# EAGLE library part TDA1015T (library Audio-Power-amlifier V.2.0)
The TDA1010A is a monolithic integrated class-B audio amplifier circuit in a 9-lead single in-line (SIL) plastic package. The device is primarily developed as a 6 W car radio amplifier for use with 4 Wand 2 Wload impedances. The wide supply voltage range and the flexibility of the IC make it an attractive proposition for record players and tape recorders with output powers up to 10 W.
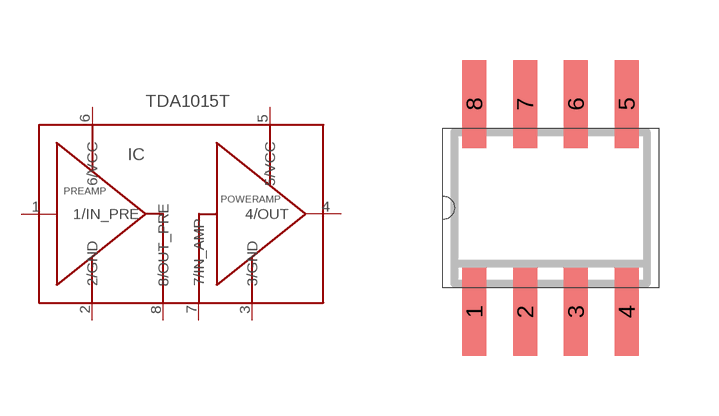
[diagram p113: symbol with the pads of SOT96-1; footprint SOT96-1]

Designator prefix IC

## TDA1015T  [SOT96-1]
1  1/IN_PRE  in
2  2/GND  pwr
3  3/GND  pwr
4  4/OUT  out
5  5/VCC  pwr
6  6/VCC  pwr
7  7/IN_AMP  in
8  8/OUT_PRE  out

## Footprint SOT96-1 (pad centres in mm)
Small Outline Narrow Plastic Gull Wing 150-mil body, package type SN
smd 0.6 x 2.2: 1 -1.905,-2.6; 2 -0.635,-2.6; 3 0.635,-2.6; 4 1.905,-2.6; 5 1.905,2.6; 6 0.635,2.6; 7 -0.635,2.6; 8 -1.905,2.6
